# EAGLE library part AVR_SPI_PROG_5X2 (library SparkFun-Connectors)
AVR 10-pin ICSP Header This is the standard AVR In Circuit Serial Programming header. Minimal, but includes pin one indicator. Works with standard Olimex programmers. SparkFun Products: 2x5 AVR ICSP Male Header - PTH 2x5 Pin Shrouded Header - PTH2
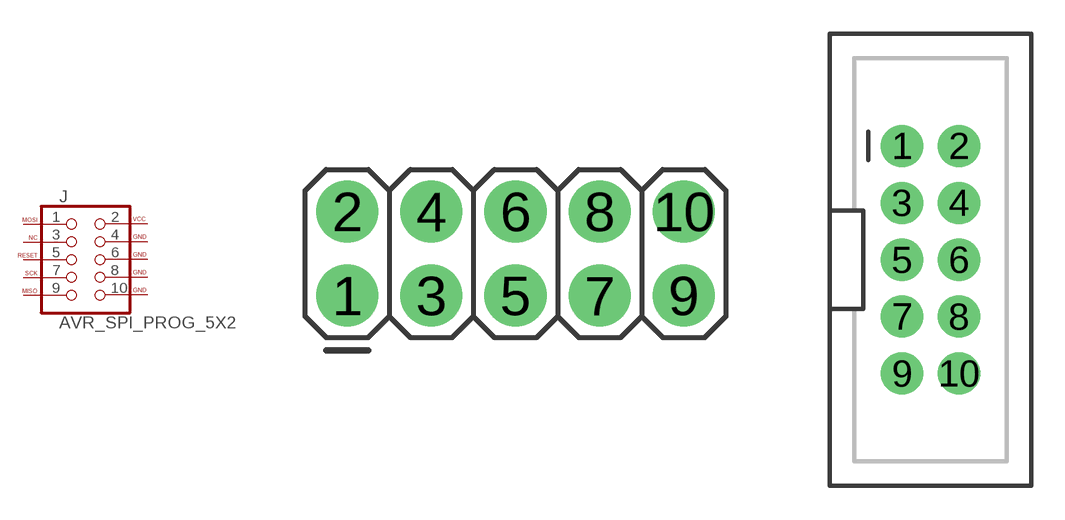
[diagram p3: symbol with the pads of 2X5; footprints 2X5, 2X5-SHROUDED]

Designator prefix J

## AVR_SPI_PROG_5X2PTH  [2X5]
1  MOSI  pas
2  VCC  pwr
3  NC  nc
4  GND  pwr
5  RESET  pas
6  GND  pwr
7  SCK  pas
8  GND  pwr
9  MISO  pas
10  GND  pwr

## AVR_SPI_PROG_5X2PTH2 (PROD_ID: CONN-08671; SF_ID: PRT-08506)  [2X5-SHROUDED]
Pads as for 2X5

## AVR_SPI_PROG_5X2LOCK (PROD_ID: CONN-08671; SF_ID: PRT-08506)  [2X5-SHROUDED_LOCK]
Pads as for 2X5

## AVR_SPI_PROG_5X2SMD  [2X5-SHROUDED_SMD]
Pads as for 2X5

## Footprint 2X5 (pad centres in mm)
Plated Through Hole - 2x5 Specifications: Pin count:10 Pin pitch:0.1" Example device(s): CONN_05x2
drill 1.016 pad 1.88: 1 0,0; 2 0,2.54; 3 2.54,0; 4 2.54,2.54; 5 5.08,0; 6 5.08,2.54; 7 7.62,0; 8 7.62,2.54; 9 10.16,0; 10 10.16,2.54

## Footprint 2X5-SHROUDED (pad centres in mm)
Plated Through Hole - 2x5 Shrouded Header Specifications: Pin count:10 Pin pitch:0.1" Datasheet referenced for footprint Example device(s): CONN_05x2
drill 1.016 pad 1.88: 1 -1.27,5.08; 2 1.27,5.08; 3 -1.27,2.54; 4 1.27,2.54; 5 -1.27,0; 6 1.27,0; 7 -1.27,-2.54; 8 1.27,-2.54; 9 -1.27,-5.08; 10 1.27,-5.08

## Footprint 2X5-SHROUDED_LOCK (pad centres in mm)
Plated Through Hole - 2x5 Shrouded Header Locking Footprint Holes are offset 0.005" from center, to hold pins in place during soldering. Specifications: Pin count:10 Pin pitch:0.1" Datasheet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
drill 1.016 pad 1.88: 1 -1.397,5.08; 2 1.397,5.08; 3 -1.397,2.54; 4 1.397,2.54; 5 -1.397,0; 6 1.397,0; 7 -1.397,-2.54; 8 1.397,-2.54; 9 -1.397,-5.08; 10 1.397,-5.08

## Footprint 2X5-SHROUDED_SMD (pad centres in mm)
Surface Mount - 2x5 Shrouded Header Specifications: Pin count:10 Pin pitch:0.1" Datasheet referenced for footprint Example device(s): CONN_05x2
smd 4.15 x 1: 1 -2.794,5.08; 2 2.794,5.08; 3 -2.794,2.54; 4 2.794,2.54; 5 -2.794,0; 6 2.794,0; 7 -2.794,-2.54; 8 2.794,-2.54; 9 -2.794,-5.08; 10 2.794,-5.08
